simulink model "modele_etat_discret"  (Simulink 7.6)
settings: Solver=ode14x  StartTime=0.0  StopTime=100  RelTol=1e-3
InitFcn:
  | clear all
  | clc
  | close all
  | b1=1;
  | b2=-0.5;
  | 
  | a1=0.2;
  | a2=-0.5;
StopFcn:
  | y=[temps sortie_etat_discret];
  | u=[temps entree_etat_discret];
  | figure(1)
  | plot(temps,entree_etat_discret)
  | title('entrée du modèle d''état')
  | xlabel('temps discret')
  | grid
  | 
  | figure(2)
  | plot(temps,sortie_etat_discret)
  | title('sortie du modèle d''état')
  | xlabel('temps discret')
  | grid
libraries: simulink x1

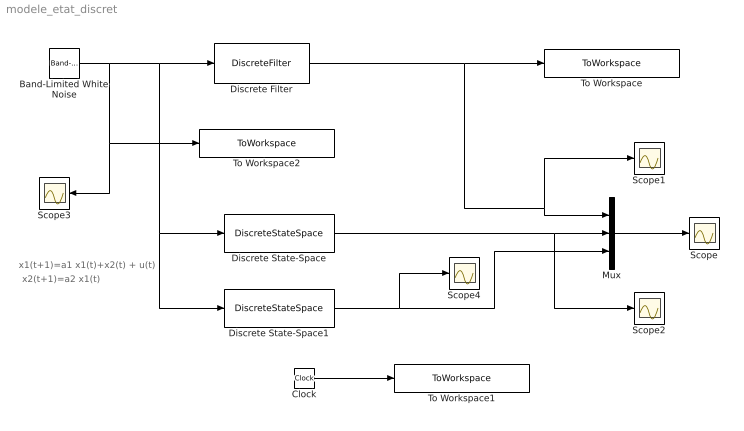
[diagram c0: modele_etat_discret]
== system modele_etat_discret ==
  note: x1(t+1)=a1 x1(t)+x2(t) + u(t)
  note: x2(t+1)=a2 x1(t)
  Band-Limited White Noise : simulink/Sources/Band-Limited White Noise  SystemSampleTime=-1  Cov=[0.1]  Ts=1  seed=[23341]
  Clock : Clock
  Discrete Filter : DiscreteFilter  Numerator="[0 b1  b2]"  Denominator=[1 -a1 -a2]  SampleTime=1
  Discrete State-Space : DiscreteStateSpace  A=[a1 1;a2 0]  B=[b1 b2]'  C=[1 0]  D=0
  Discrete State-Space1 : DiscreteStateSpace  A=|  B=|  C="[3.2955      -2.4554]"  D=0
      | [0.19452     -0.51151
      |     ;   0.97542    0.0054797]
      | [0.24588;
      |  -0.077257]
  Mux : Mux  Inputs=3
  Scope{,1..4} (5 alike) : Scope
  To Workspace : ToWorkspace  VariableName=sortie_etat_discret  SampleTime=-1  SaveFormat=Array
  To Workspace1 : ToWorkspace  VariableName=temps  SampleTime=-1  SaveFormat=Array
  To Workspace2 : ToWorkspace  VariableName=entree_etat_discret  SampleTime=-1  SaveFormat=Array
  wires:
  Band-Limited White Noise/1 -> Discrete Filter/1, Discrete State-Space/1, Discrete State-Space1/1, To Workspace2/1, Scope3/1
  Discrete Filter/1 -> To Workspace/1, Mux/1, Scope1/1
  Discrete State-Space/1 -> Mux/2, Scope2/1
  Mux/1 -> Scope/1
  Clock/1 -> To Workspace1/1
  Discrete State-Space1/1 -> Mux/3, Scope4/1
